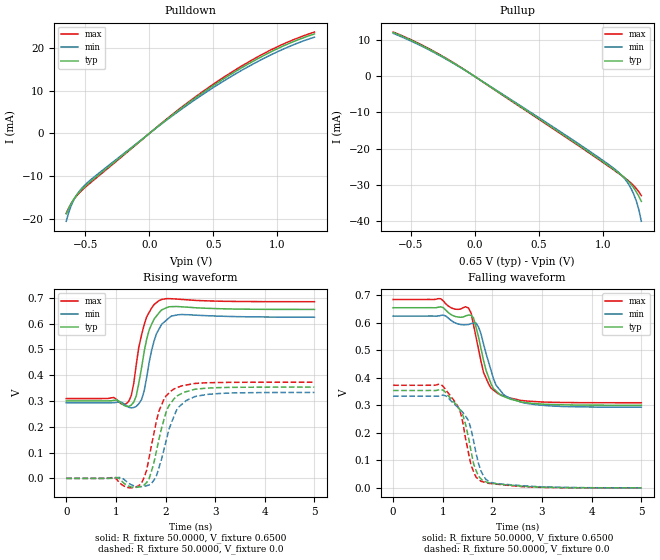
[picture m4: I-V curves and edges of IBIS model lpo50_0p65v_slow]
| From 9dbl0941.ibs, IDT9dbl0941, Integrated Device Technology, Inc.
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|   Model lpo50_0p65v_slow
[Model]  lpo50_0p65v_slow
Model_type Output
Polarity   Non-Inverting
Vmeas =  0.4000V
Cref =   2.0000pF
Rref =   0.0
Vref =   0.4000V
C_comp   1.1000pF   1.0000pF   1.2000pF
[Temperature Range]   27.0000   70.0000   0.0
[Voltage Range]   0.6500V   0.6200V   0.6800V
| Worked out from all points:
|   slope of the pulldown table from 0 to 0.098 V, typ, clamps not added: 41.2 ohm
|   slope of the pullup table from 0 to 0.098 V, typ, clamps not added: 43 ohm
|   rising waveform, R_fixture 50.0000, V_fixture 0.6500: 20-80 % time 226ps typ, 225ps min, 222ps max; typ from 0.3 V to 0.655 V
|   rising waveform, R_fixture 50.0000, V_fixture 0.0: 20-80 % time 295ps typ, 322ps min, 286ps max; typ from 0 V to 0.354 V
|   falling waveform, R_fixture 50.0000, V_fixture 0.6500: 20-80 % time 321ps typ, 363ps min, 307ps max; typ from 0.655 V to 0.3 V
|   falling waveform, R_fixture 50.0000, V_fixture 0.0: 20-80 % time 307ps typ, 324ps min, 292ps max; typ from 0.354 V to 0 V
[Pulldown]
|Voltage   I(typ)   I(min)   I(max)
-650mV    -18.76mA   -20.5mA    -18.62mA
-630mV    -17.42mA   -18.38mA   -17.37mA
-610mV    -16.28mA   -16.76mA   -16.29mA
-590mV    -15.29mA   -15.48mA   -15.38mA
-550mV    -13.73mA   -13.58mA   -13.94mA
-510mV    -12.53mA   -12.21mA   -12.79mA
-390mV    -9.514mA   -9.154mA   -9.768mA
170mV     4.068mA    3.887mA    4.195mA
470mV     10.56mA    10.12mA    10.87mA
770mV     16.15mA    15.52mA    16.57mA
1.03V     20.16mA    19.44mA    20.62mA
1.29V     23.19mA    22.45mA    23.64mA
[Pullup]
|Voltage   I(typ)   I(min)   I(max)
-640mV    11.97mA    11.72mA    12.07mA
-400mV    8.099mA    7.887mA    8.218mA
-140mV    2.942mA    2.851mA    3.002mA
660mV     -15.52mA   -15.2mA    -15.71mA
1.08V     -25.64mA   -25.34mA   -25.8mA
1.16V     -27.78mA   -27.91mA   -27.83mA
1.2V      -29.1mA    -29.81mA   -28.92mA
1.22V     -29.9mA    -31.04mA   -29.53mA
1.24V     -30.83mA   -32.53mA   -30.21mA
1.26V     -31.91mA   -34.39mA   -31mA
1.28V     -33.14mA   -36.79mA   -31.92mA
1.3V      -34.56mA   -40.04mA   -32.99mA
[Ramp]
| variable   typ   min   max
dV/dt_r  0.2123/0.2953n   0.1999/0.3220n   0.2237/0.2858n
dV/dt_f  0.2127/0.3213n   0.1989/0.3633n   0.2252/0.3074n
R_load = 50.0000
[Rising Waveform]
R_fixture= 50.0000
V_fixture= 0.6500
V_fixture_min= 0.6200
V_fixture_max= 0.6800
|time   V(typ)   V(min)   V(max)
0s        300.2mV    293mV      309.4mV
1.01ns    304.2mV    294.6mV    306.7mV
1.26ns    279.5mV    275.7mV    299.2mV
1.31ns    284.2mV    273.6mV    320.8mV
1.41ns    319.6mV    279.1mV    440.2mV
1.57ns    491.6mV    339.5mV    596.2mV
1.72ns    597.6mV    496.5mV    660.3mV
1.92ns    652.8mV    596.8mV    693.5mV
2.27ns    665.7mV    634.7mV    694.5mV
5ns       654.9mV    624.8mV    684.9mV
[Rising Waveform]
R_fixture= 50.0000
V_fixture= 0.0
V_fixture_min= 0.0
V_fixture_max= 0.0
|time   V(typ)   V(min)   V(max)
0s        731.2nV    0V         944.6nV
1.11ns    -8.888mV   2.904mV    -22.89mV
1.46ns    -33.2mV    -32.18mV   -28.15mV
1.67ns    -484.6uV   -25.26mV   81.65mV
1.82ns    109mV      12.06mV    225.5mV
1.97ns    228.7mV    113.2mV    308.3mV
2.12ns    295.1mV    216.4mV    340.1mV
2.32ns    328.6mV    285.6mV    358.4mV
2.88ns    350.3mV    326.2mV    370.8mV
5ns       353.8mV    333.2mV    372.9mV
[Falling Waveform]
R_fixture= 50.0000
V_fixture= 0.6500
V_fixture_min= 0.6200
V_fixture_max= 0.6800
|time   V(typ)   V(min)   V(max)
0s        654.8mV    624.6mV    684.8mV
1.01ns    655mV      627.9mV    679.7mV
1.52ns    628.5mV    593.8mV    653.3mV
1.62ns    617.8mV    598.9mV    592.1mV
1.72ns    548.5mV    584.7mV    504.3mV
1.82ns    463.9mV    523.7mV    420.3mV
1.97ns    379.4mV    428.6mV    363mV
2.12ns    344.7mV    362.9mV    341.6mV
2.88ns    306mV      302.2mV    313.4mV
5ns       300.3mV    293.1mV    309.4mV
[Falling Waveform]
R_fixture= 50.0000
V_fixture= 0.0
V_fixture_min= 0.0
V_fixture_max= 0.0
|time   V(typ)   V(min)   V(max)
0s        353.9mV    333.3mV    372.9mV
1.01ns    354.9mV    337.1mV    368.4mV
1.36ns    279.9mV    282.7mV    272.2mV
1.41ns    261.6mV    272.8mV    232.4mV
1.52ns    182mV      244mV      125.4mV
1.62ns    88.33mV    171.9mV    59.15mV
1.77ns    32.68mV    60.9mV     23.99mV
1.87ns    21.7mV     30.27mV    18.97mV
2.17ns    12.95mV    13.95mV    11.69mV
5ns       18.66uV    54.1uV     8.023uV
